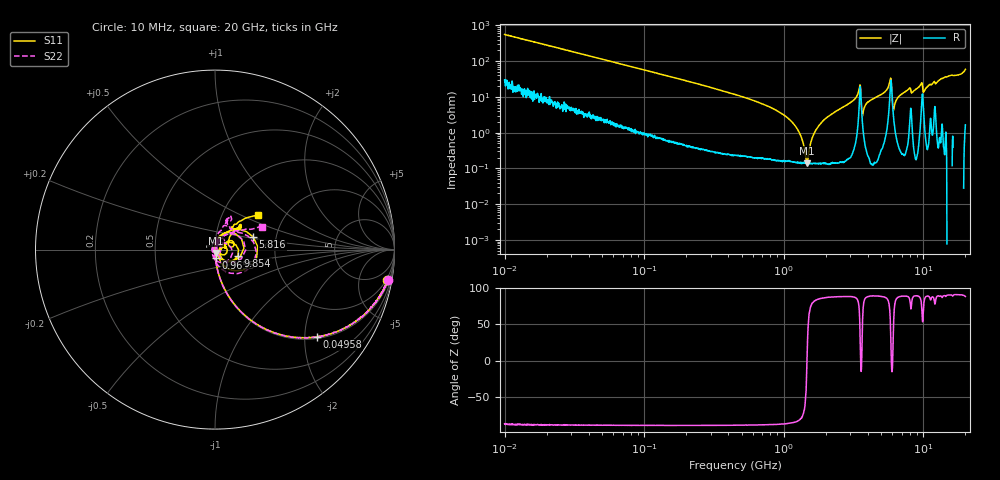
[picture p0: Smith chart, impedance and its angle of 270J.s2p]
!Keysight Technologies,P5008B,MY61100088,A.16.20.02
!Date: Tuesday, November 07, 2023 15:53:20
!Correction: S11(C  2-Port  )
!S21(C  2-Port  )
!S12(C  2-Port  )
!S22(C  2-Port  )
!S2P File: Measurements: S11, S21, S12, S22:Log Frequency Sweep
# Hz S  dB  R 50
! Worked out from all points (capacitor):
!   1601 points, 10 MHz to 20 GHz, reference 50 ohm
!   read as one part in series: C = 28.3 pF near 10.39 MHz
!   lowest |Z| = 139 mohm at 1.467 GHz (marker M1)
!   series resonance near 1.466 GHz, so ESL is about 420 pH
!   S11 on the Smith chart (normalised r, x): 10 MHz: 2, -11; 49.58 MHz: 1.04, -2.30; 965.5 MHz: 1.00, -0.09; 5.816 GHz: 1.52, +0.23; 9.854 GHz: 1.29, -0.09; 20 GHz: 1.47, +0.63
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1e7  -0.21 -10.0  -15.19 77.0  -15.19 77.0  -0.21 -10.0
3.555162e7  -1.53 -31.7  -5.59 56.9  -5.59 56.9  -1.53 -31.8
4.957691e7  -2.53 -40.5  -3.75 48.3  -3.75 48.3  -2.53 -40.6
1.263918e8  -7.73 -65.0  -0.86 24.0  -0.87 24.0  -7.73 -65.1
4.472136e8  -18.23 -82.3  -0.09 6.3  -0.09 6.3  -18.23 -82.8
9.654822e8  -26.61 -85.2  -0.02 1.3  -0.03 1.3  -26.59 -88.2
1.466564e9  -34.39 -80.0  -0.01 -1.1  -0.01 -1.1  -34.41 -93.3
1.589917e9  -36.92 -76.6  -0.01 -1.6  -0.01 -1.6  -37.02 -94.9
1.842179e9  -43.09 -60.1  -0.01 -2.5  -0.01 -2.4  -43.88 -99.9
2.09429e9  -48.79 8.5  -0.01 -3.3  -0.01 -3.3  -64.50 171.0
2.347211e9  -42.91 71.6  -0.01 -4.1  -0.01 -4.1  -44.11 71.6
3.44879e9  -20.06 62.9  -0.35 -11.0  -0.35 -11.0  -19.82 53.8
3.865292e9  -43.23 100.7  -0.03 -6.7  -0.03 -6.7  -38.73 22.1
5.652411e9  -18.86 57.2  -0.35 -16.9  -0.35 -16.8  -18.80 51.0
5.815842e9  -13.00 18.3  -1.84 -17.7  -1.84 -17.7  -13.19 10.5
6.738606e9  -30.95 -22.8  -0.01 -12.6  -0.01 -12.6  -36.23 179.3
7.844959e9  -25.47 25.9  -0.04 -17.1  -0.04 -17.0  -28.25 97.9
8.709232e9  -32.57 -9.2  0.01 -18.2  0.01 -18.2  -38.21 146.9
9.854205e9  -17.58 -14.8  -1.00 -20.1  -1.00 -20.1  -20.07 -31.9
1.063241e10  -30.24 -8.1  0.00 -22.0  -0.00 -21.9  -35.93 140.8
1.374174e10  -15.85 42.1  -0.15 -29.7  -0.16 -29.6  -16.42 67.2
2e10  -10.21 38.8  -0.65 -54.8  -0.65 -54.7  -10.64 25.9
